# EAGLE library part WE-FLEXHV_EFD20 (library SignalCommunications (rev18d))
WE-FLEX HV Flexible Transformer for DC/DC Converter Characteristics Transformer with 6 identical windings 4 sizes with 5 different lengths of air gap each Isolation voltage up to 1.5 kVAC Low leakage inductance Operating temperature: –40 ºC to +125 ºC By using different circuits more than 375 transformer solutions and about 125 choke solutions possible. Consequently, quick prototyping possibilities EFD size parts provide Basic insulation for a working voltage of 250VRMS when they are connteced approbiate Applications Flyback converters Forward converters Push-pull converters Step-up/step-down converters SEPIC Details see: http://katalog.we-online.de/en/pbs/WE-FLEXHV/749196308?m Created by Yingchun Shan 2017 (C) Wurth Elektronik
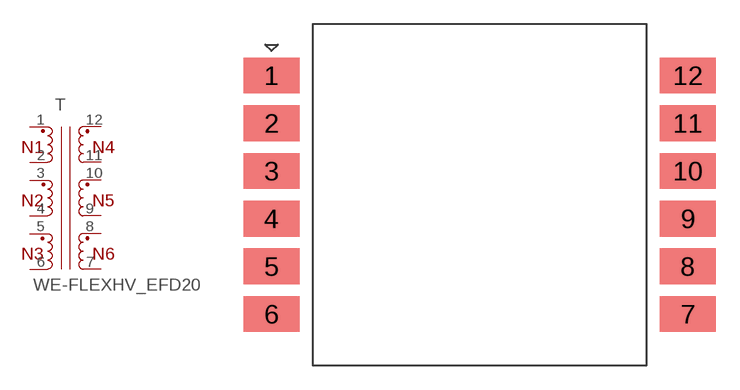
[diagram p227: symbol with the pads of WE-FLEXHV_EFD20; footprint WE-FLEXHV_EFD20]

Designator prefix T

## WE-FLEXHV_EFD20_749196507 (WE-NUMBER: 749196507/0,18uH), WE-FLEXHV_EFD20_749196508 (WE-NUMBER: 749196508/0,24uH), WE-FLEXHV_EFD20_749196517 (WE-NUMBER: 749196517/0,18uH), WE-FLEXHV_EFD20_749196518 (WE-NUMBER: 749196518/0,24uH), WE-FLEXHV_EFD20_749196527 (WE-NUMBER: 749196527/0,18uH), WE-FLEXHV_EFD20_749196528 (WE-NUMBER: 749096528/0,24uH), WE-FLEXHV_EFD20_749196537 (WE-NUMBER: 749196537/0,18uH), WE-FLEXHV_EFD20_749196538 (WE-NUMBER: 749196538/0,24uH), WE-FLEXHV_EFD20_749196547 (WE-NUMBER: 749196547/0,18uH), WE-FLEXHV_EFD20_749196548 (WE-NUMBER: 749196548/0,24uH)  [WE-FLEXHV_EFD20]
1  1  pas
2  2  pas
3  3  pas
4  4  pas
5  5  pas
6  6  pas
7  7  pas
8  8  pas
9  9  pas
10  10  pas
11  11  pas
12  12  pas

## Footprint WE-FLEXHV_EFD20 (pad centres in mm)
smd 3.5 x 2.25: 1 -13.1,7.5; 2 -13.1,4.5; 3 -13.1,1.5; 4 -13.1,-1.5; 5 -13.1,-4.5; 6 -13.1,-7.5; 7 13.1,-7.5; 8 13.1,-4.5; 9 13.1,-1.5; 10 13.1,1.5; 11 13.1,4.5; 12 13.1,7.5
